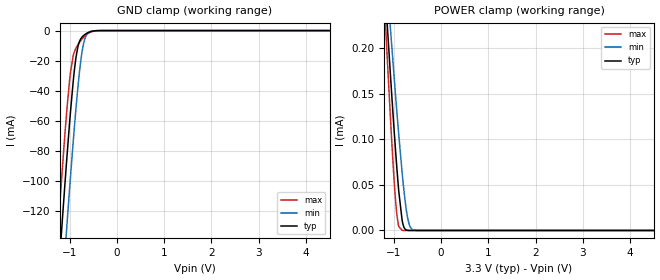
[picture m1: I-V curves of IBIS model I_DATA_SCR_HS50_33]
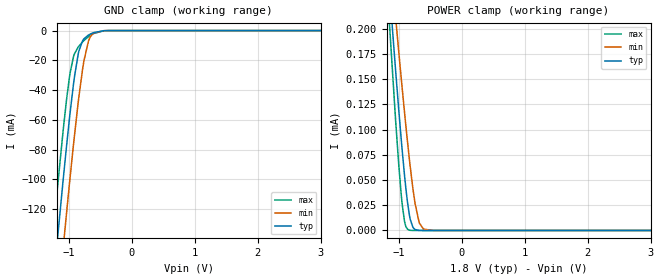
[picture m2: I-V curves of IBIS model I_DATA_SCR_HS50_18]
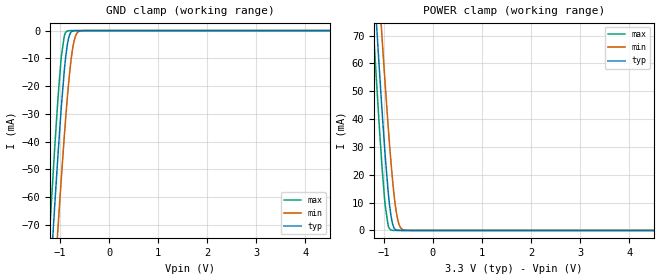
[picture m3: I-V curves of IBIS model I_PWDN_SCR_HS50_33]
| Texas Instruments Incorporated
| DS92LV2421
| 10 to 75MHz 24-bit Channel Link II Serializer
| Marketing part#   Voltage Range   Package-type   Temperature
| DS92LV2421SQE   1.71V - 3.6V   48-Pin LLP   -40 to 105C
| DS92LV2421SQ   1.71V - 3.6V   48-Pin LLP   -40 to 105C
| DS92LV2421SQX   1.71V - 3.6V   48-Pin LLP   -40 to 105C
[IBIS Ver]   4.0
[File name]   ds92lv2421.ibs
[File Rev]   1.0
[Date]   03/26/2012
[Source]   Model built from TISPICE simulations at:
   Texas Instruments Incorporated.
   WEBENCH DESIGN CENTER
   12500 TI Blvd
   Dallas, TX -75243
   For Support e-mail: elab_scm_ibis@list.ti.com
[Notes]   Rev 1.0: 03/26/2012
   - Initial version of the IBIS model
   - All models are generated in Spectre
   - ccomp is listed in numerical order, for PVT information,
   please check notes above ccomp keyword for each model
   - All non-monotonic warnings can be ignored as per buffer behavior
[Disclaimer] This product is designed as an aid for customers of Texas Instruments.
   No warranties, either expressed or implied, with respect to this third
   party software (if any) or with respect to its fitness for any
   particular purpose is claimed by Texas Instruments or the author. The
   software (if any) is provided solely on an "as is" basis. The entire
   risk as to its quality and performance is with the customer
[Copyright]   (C)Copyright 2012 Texas Instruments Incorporated.
   All rights reserved.
|   DS92LV2421
[Component]   DS92LV2421
[Manufacturer]  Texas Instruments, Inc.
[Package]   |48-pin LLP 7.0X7.0X0.8mm
|   typ   min   max
R_pkg   0   0   0
L_pkg   0   0   0
C_pkg   0   0   0
[Pin]   signal_name   model_name   R_pin   L_pin   C_pin
1   DI22   I_DATA_SCR_HS50
2   DI23   I_DATA_SCR_HS50
3   CI2   I_DATA_SCR_HS50
4   CI3   I_DATA_SCR_HS50
5   CI1   I_DATA_MC_HS50
6   ID[x]   NC
7   VDDL   POWER
8   SCL   IO_SMBUS_HS50
9   SDA   IO_SMBUS_HS50
10   CLKIN   I_CLK_HS50
11   RFB   I_DATA_SCR_HS50
12   CONFIG[0]   I_DATA_SCR_HS50
13   CONFIG[1]   I_DATA_SCR_HS50
14   VDDP   POWER
15   RES0   NC
16   RES1   NC
17   VDDHS   POWER
18   RES2   NC
19   DOUT-   NC
20   DOUT+   NC
21   PDB   I_PWDN_SCR_HS50
22   VDDTX   POWER
23   DeEmph   NC
24   VODSEL   I_DATA_SCR_HS50
25   DI0   I_DATA_SCR_HS50
26   DI1   I_DATA_SCR_HS50
27   DI2   I_DATA_SCR_HS50
28   DI3   I_DATA_SCR_HS50
29   DI4   I_DATA_SCR_HS50
30   VDDIO   POWER
31   BISTEN   I_DATA_SCR_HS50
32   DI5   I_DATA_SCR_HS50
33   DI6   I_DATA_SCR_HS50
34   DI7   I_DATA_SCR_HS50
35   DI8   I_DATA_SCR_HS50
36   DI9   I_DATA_SCR_HS50
37   DI10   I_DATA_SCR_HS50
38   DI11   I_DATA_SCR_HS50
39   DI12   I_DATA_SCR_HS50
40   DI13   I_DATA_SCR_HS50
41   DI14   I_DATA_SCR_HS50
42   DI15   I_DATA_SCR_HS50
43   DI16   I_DATA_SCR_HS50
44   DI17   I_DATA_SCR_HS50
45   DI18   I_DATA_SCR_HS50
46   DI19   I_DATA_SCR_HS50
47   DI20   I_DATA_SCR_HS50
48   DI21   I_DATA_SCR_HS50
49   DAP   GND
[Package Model]  llp48_ds90ur905
[Diff pin]  inv_pin  vdiff  tdelay_typ  tdelay_min  tdelay_max
20   19   0.0   0.0s   0.0s   0.0s
[Model Selector]   I_DATA_SCR_HS50
I_DATA_SCR_HS50_33   I_DATA_SCR_HS50 input with VDD=3.3V
I_DATA_SCR_HS50_18   I_DATA_SCR_HS50 input with VDD=1.8V
[Model Selector]   I_DATA_MC_HS50
I_DATA_MC_HS50_33   I_DATA_MC_HS50 input with VDD=3.3V
I_DATA_MC_HS50_18   I_DATA_MC_HS50 input with VDD=1.8V
[Model Selector]   I_CLK_HS50
I_CLK_HS50_33   I_CLK_HS50 with VDD=3.3V
I_CLK_HS50_18   I_CLK_HS50 with VDD=1.8V
[Model Selector]   I_PWDN_SCR_HS50
I_PWDN_SCR_HS50_33   I_PWDN_SCR_HS50 input with VDD=3.3V
I_PWDN_SCR_HS50_18   I_PWDN_SCR_HS50 input with VDD=1.8V
[Model Selector]   IO_SMBUS_HS50
IO_SMBUS_HS50_33   IO_SMBUS_HS50 with VDD=3.3V
IO_SMBUS_HS50_18   IO_SMBUS_HS50 with VDD=1.8V
[Define Package Model]  llp48_ds90ur905
[Manufacturer]  Texas Instruments, Inc.
[OEM]  Texas Instruments, Inc.
[Description] 7.0x7.0x0.8mm 48-pin LLP
[Number Of Pins]  49
[Pin Numbers]
49   | 49 = DAP
1   | 1 = L1
2   | 2 = L2
3   | 3 = L3
4   | 4 = L4
5   | 5 = L5
6   | 6 = L6
7   | 7 = L7
8   | 8 = L8
9   | 9 = L9
10   | 10 = L10
11   | 11 = L11
12   | 12 = L12
13   | 13 = L13
14   | 14 = L14
15   | 15 = L15
16   | 16 = L16
17   | 17 = L17
18   | 18 = L18
19   | 19 = L19
20   | 20 = L20
21   | 21 = L21
22   | 22 = L22
23   | 23 = L23
24   | 24 = L24
25   | 25 = L25
26   | 26 = L26
27   | 27 = L27
28   | 28 = L28
29   | 29 = L29
30   | 30 = L30
31   | 31 = L31
32   | 32 = L32
33   | 33 = L33
34   | 34 = L34
35   | 35 = L35
36   | 36 = L36
37   | 37 = L37
38   | 38 = L38
39   | 39 = L39
40   | 40 = L40
41   | 41 = L41
42   | 42 = L42
43   | 43 = L43
44   | 44 = L44
45   | 45 = L45
46   | 46 = L46
47   | 47 = L47
48   | 48 = L48
[Model Data]
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[End Model Data]
[End Package Model]
| Models and submodels in the file (10): I_DATA_SCR_HS50_33 (Input), I_DATA_SCR_HS50_18 (Input), I_CLK_HS50_33 (Input), I_CLK_HS50_18 (Input), I_PWDN_SCR_HS50_33 (Input), I_PWDN_SCR_HS50_18 (Input), I_DATA_MC_HS50_18 (Input), I_DATA_MC_HS50_33 (Input), IO_SMBUS_HS50_33 (I/O_open_drain), IO_SMBUS_HS50_18 (I/O_open_drain)
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|   Model I_DATA_SCR_HS50_33
[Model] I_DATA_SCR_HS50_33
Model_type Input
Vinl =   0.8
Vinh =   2.0
|   typ   min   max
|   (nom)   (slow)   (fast)
C_comp   0.3665pF   0.3665pF   0.3665pF
[Temperature Range]   25.000   105.000   -40.000
[Voltage Range]   3.300V   3.0000V   3.6000V
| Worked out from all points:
|   GND clamp passes 1 mA (typ) near -0.58 V on its own axis
|   POWER clamp passes 1 mA (typ) near -2.02 V on its own axis
[GND Clamp]
|   Voltage   I(typ)   I(min)   I(max)
-3.3V     -1.166A    -1.209A    -1.134A
-1.32V    -202.1mA   -249mA     -167.1mA
-1.241V   -165.6mA   -212.4mA   -130.7mA
-1.142V   -121mA     -167.4mA   -86.89mA
-1.063V   -86.78mA   -132.3mA   -54.56mA
-983.4mV  -54.93mA   -98.36mA   -28.27mA
-924mV    -33.98mA   -74.16mA   -16.74mA
-825mV    -10.8mA    -38mA      -9.446mA
-755.7mV  -5.134mA   -18.34mA   -6.356mA
-696.3mV  -3.098mA   -7.601mA   -4.22mA
-567.6mV  -815.5uA   -746uA     -1.217mA
6.59V     0A         0A         0A
[POWER Clamp]
|   Voltage   I(typ)   I(min)   I(max)
-3.3V     2.159mA    1.892mA    2.559mA
-1.191V   270.3uA    306.6uA    243.1uA
-1.132V   220.6uA    264.4uA    182.9uA
-1.063V   164.1uA    216.1uA    115.7uA
-993.3mV  110.2uA    168.9uA    55.28uA
-933.9mV  67.72uA    129.8uA    16.89uA
-894.3mV  42.8uA     104.8uA    4.336uA
-825mV    11.61uA    64.2uA     166.8nA
-755.7mV  1.271uA    30.48uA    2.122nA
-696.3mV  130.3nA    11.15uA    0A
-557.7mV  0A         260.4nA    0A
6.59V     0A         0A         0A
|   Model I_DATA_SCR_HS50_18
[Model] I_DATA_SCR_HS50_18
Model_type Input
Vinl =   0.63
Vinh =   1.17
|   typ   min   max
|   (nom)   (fast)   (slow)
C_comp   0.5298pF   0.3665pF   0.5298pF
[Temperature Range]   25.000   105.000   -40.000
[Voltage Range]   1.800V   1.7100V   1.8900V
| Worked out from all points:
|   GND clamp passes 1 mA (typ) near -0.56 V on its own axis
[GND Clamp]
|   Voltage   I(typ)   I(min)   I(max)
-1.8V     -430.9mA   -477mA     -396.6mA
-1.238V   -164.5mA   -211.3mA   -129.6mA
-1.174V   -135.2mA   -181.7mA   -100.7mA
-1.093V   -99.54mA   -145.4mA   -66.37mA
-1.039V   -76.81mA   -121.8mA   -45.69mA
-984.6mV  -55.39mA   -98.86mA   -28.59mA
-930.6mV  -36.12mA   -76.78mA   -17.61mA
-855mV    -15.77mA   -48.21mA   -11.06mA
-763.2mV  -5.498mA   -20.14mA   -6.658mA
-687.6mV  -2.877mA   -6.556mA   -3.945mA
-450mV    -97.64uA   -77.9uA    -176.8uA
3.595V    0A         0A         0A
[POWER Clamp]
|   Voltage   I(typ)   I(min)   I(max)
-1.8V     803.7uA    754.7uA    897.4uA
-1.157V   241.8uA    282.5uA    208.5uA
-1.055V   157.9uA    210.7uA    108.4uA
-1.012V   124.1uA    181.2uA    70.17uA
-952.2mV  80.3uA     141.7uA    26.6uA
-914.4mV  55uA       117.4uA    9.25uA
-865.8mV  27.6uA     87.52uA    1.228uA
-822.6mV  10.92uA    62.89uA    149.1nA
-747mV    921.8nA    26.99uA    1.513nA
-682.2mV  75.41nA    8.215uA    0A
-612mV    3.441nA    1.296uA    0A
3.595V    0A         0A         0A
|   Model I_PWDN_SCR_HS50_33
[Model] I_PWDN_SCR_HS50_33
Model_type Input
Vinl =   0.8
Vinh =   2.0
|   typ   min   max
|   (nom)   (fast)   (slow)
C_comp   0.3665pF   0.3665pF   0.5298pF
[Temperature Range]   25.000   105.000   -40.000
[Voltage Range]   3.300V   3.0000V   3.6000V
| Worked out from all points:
|   GND clamp passes 1 mA (typ) near -0.79 V on its own axis
|   POWER clamp passes 1 mA (typ) near -0.79 V on its own axis
[GND Clamp]
|   Voltage   I(typ)   I(min)   I(max)
-3.3V     -740.6mA   -745.8mA   -738.2mA
-1.211V   -92.27mA   -118mA     -71.83mA
-1.191V   -86.5mA    -112.3mA   -65.95mA
-1.112V   -63.85mA   -90.11mA   -43.04mA
-1.043V   -44.84mA   -71.14mA   -24.45mA
-973.5mV  -27.25mA   -52.87mA   -9.257mA
-914.1mV  -14.38mA   -38.09mA   -1.938mA
-854.7mV  -5.279mA   -24.66mA   -158.3uA
-785.4mV  -769.6uA   -11.9mA    -11.81uA
-726mV    -91.41uA   -4.691mA   -6.467uA
-577.5mV  -3.449uA   -99.25uA   -4.919uA
6.59V     0A         0A         0A
[POWER Clamp]
|   Voltage   I(typ)   I(min)   I(max)
-3.3V     739mA      744.2mA    736.5mA
-1.211V   92.02mA    117.6mA    71.62mA
-1.191V   86.27mA    112mA      65.75mA
-1.112V   63.66mA    89.86mA    42.89mA
-1.043V   44.7mA     70.93mA    24.36mA
-973.5mV  27.14mA    52.7mA     9.21mA
-914.1mV  14.31mA    37.95mA    1.931mA
-854.7mV  5.248mA    24.55mA    164.4uA
-785.4mV  767.3uA    11.83mA    19.72uA
-726mV    94.5uA     4.66mA     14.93uA
-577.5mV  8.162uA    100.4uA    14.65uA
6.59V     0A         0A         0A
